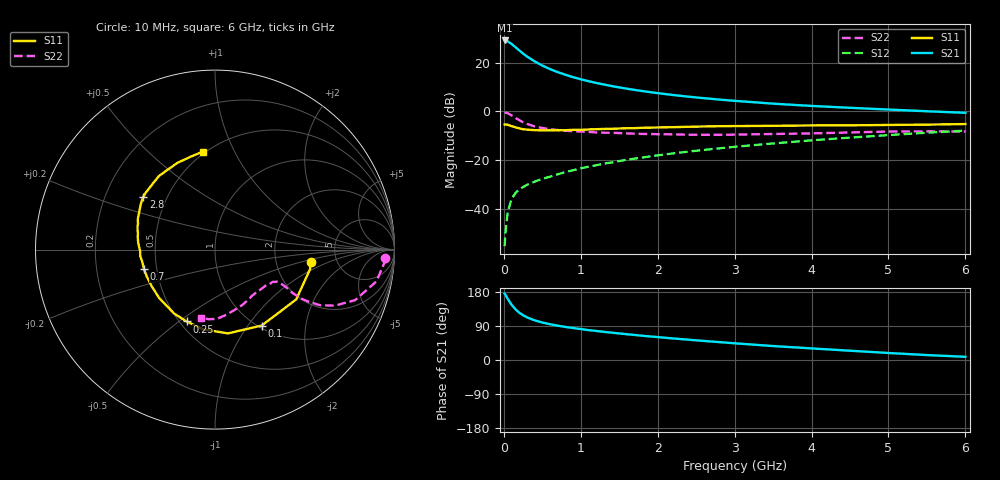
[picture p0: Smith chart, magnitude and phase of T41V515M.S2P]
! Infineon Technologies  Discrete & RF Semiconductors
! BFR182T
! Si NPN RF Bipolar Junction Transistor in SC75
! VCE = 1.5 V  IC = 15 mA
! Common Emitter S-Parameters:  October  1999
# GHz  S  MA  R  50
!  f  S11  S21  S12  S22
! GHz  MAG  ANG  MAG  ANG  MAG  ANG  MAG  ANG
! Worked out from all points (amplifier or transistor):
!   36 points, 10 MHz to 6 GHz, reference 50 ohm
!   highest |S21| = 29.2 dB at 10 MHz (marker M1)
!   |S21| within 3 dB of that: start of sweep to 159.6 MHz
!   unconditionally stable (mu >= 1): 591 MHz to 3.955 GHz
!   at 250 MHz: K = 0.63, MSG = 27.4 dB, |S12| = -31.1 dB
!   at 1.4 GHz: K = 1.17, MAG = 13.2 dB, |S12| = -21.0 dB
!   at 6 GHz: K = 0.87, MSG = 3.7 dB, |S12| = -7.9 dB
!   S11 on the Smith chart (normalised r, x): 10 MHz: 3.18, -0.64; 100 MHz: 1.04, -1.17; 250 MHz: 0.54, -0.53; 700 MHz: 0.42, -0.11; 2.8 GHz: 0.37, +0.29; 6 GHz: 0.48, +0.76
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0.01  0.5373 -7.6  28.71 175.3  0.0017 86.4  0.9457 -3.0
0.02  0.5407 -11.6  28.63 172.7  0.0031 89.7  0.9465 -4.5
0.05  0.5309 -31.5  27.57 161.5  0.0085 83.2  0.9169 -11.1
0.1  0.4968 -58.4  24.37 146.1  0.0159 69.3  0.8305 -19.8
0.15  0.4723 -81.2  20.94 133.9  0.0208 63.6  0.7368 -25.1
0.2  0.4496 -98.3  17.94 124.9  0.0254 60.5  0.6614 -27.9
0.25  0.4304 -111.5  15.45 118.1  0.0278 58.8  0.5988 -29.1
0.3  0.4229 -122.6  13.48 112.7  0.031 58.5  0.555 -29.6
0.4  0.4117 -138.8  10.67 104.6  0.036 59.1  0.4912 -29.2
0.5  0.4077 -149.5  8.766 99.0  0.0411 61.0  0.4563 -28.1
0.6  0.4085 -158.0  7.394 94.4  0.0455 62.3  0.4318 -27.6
0.7  0.4105 -164.6  6.425 90.6  0.051 64.3  0.4142 -27.3
0.9  0.4178 -175.0  5.056 84.4  0.0617 66.2  0.391 -27.3
1.1  0.4254 176.9  4.183 78.9  0.0729 67.8  0.3786 -28.4
1.3  0.4366 170.5  3.572 74.3  0.0845 68.6  0.3659 -30.0
1.6  0.4514 162.9  2.927 68.0  0.1017 69.1  0.3529 -33.0
2.2  0.4742 152.4  2.173 56.9  0.1372 68.9  0.3373 -41.6
2.8  0.4963 143.5  1.751 47.2  0.1739 67.3  0.3297 -51.4
3.5  0.505 133.5  1.443 36.8  0.2195 64.7  0.3434 -63.2
4.5  0.5174 120.7  1.186 24.5  0.2893 59.2  0.369 -80.4
5.5  0.5346 104.9  1.007 13.0  0.3646 52.5  0.3893 -95.0
6  0.5498 97.2  0.935 8.4  0.4033 48.3  0.3866 -101.4
